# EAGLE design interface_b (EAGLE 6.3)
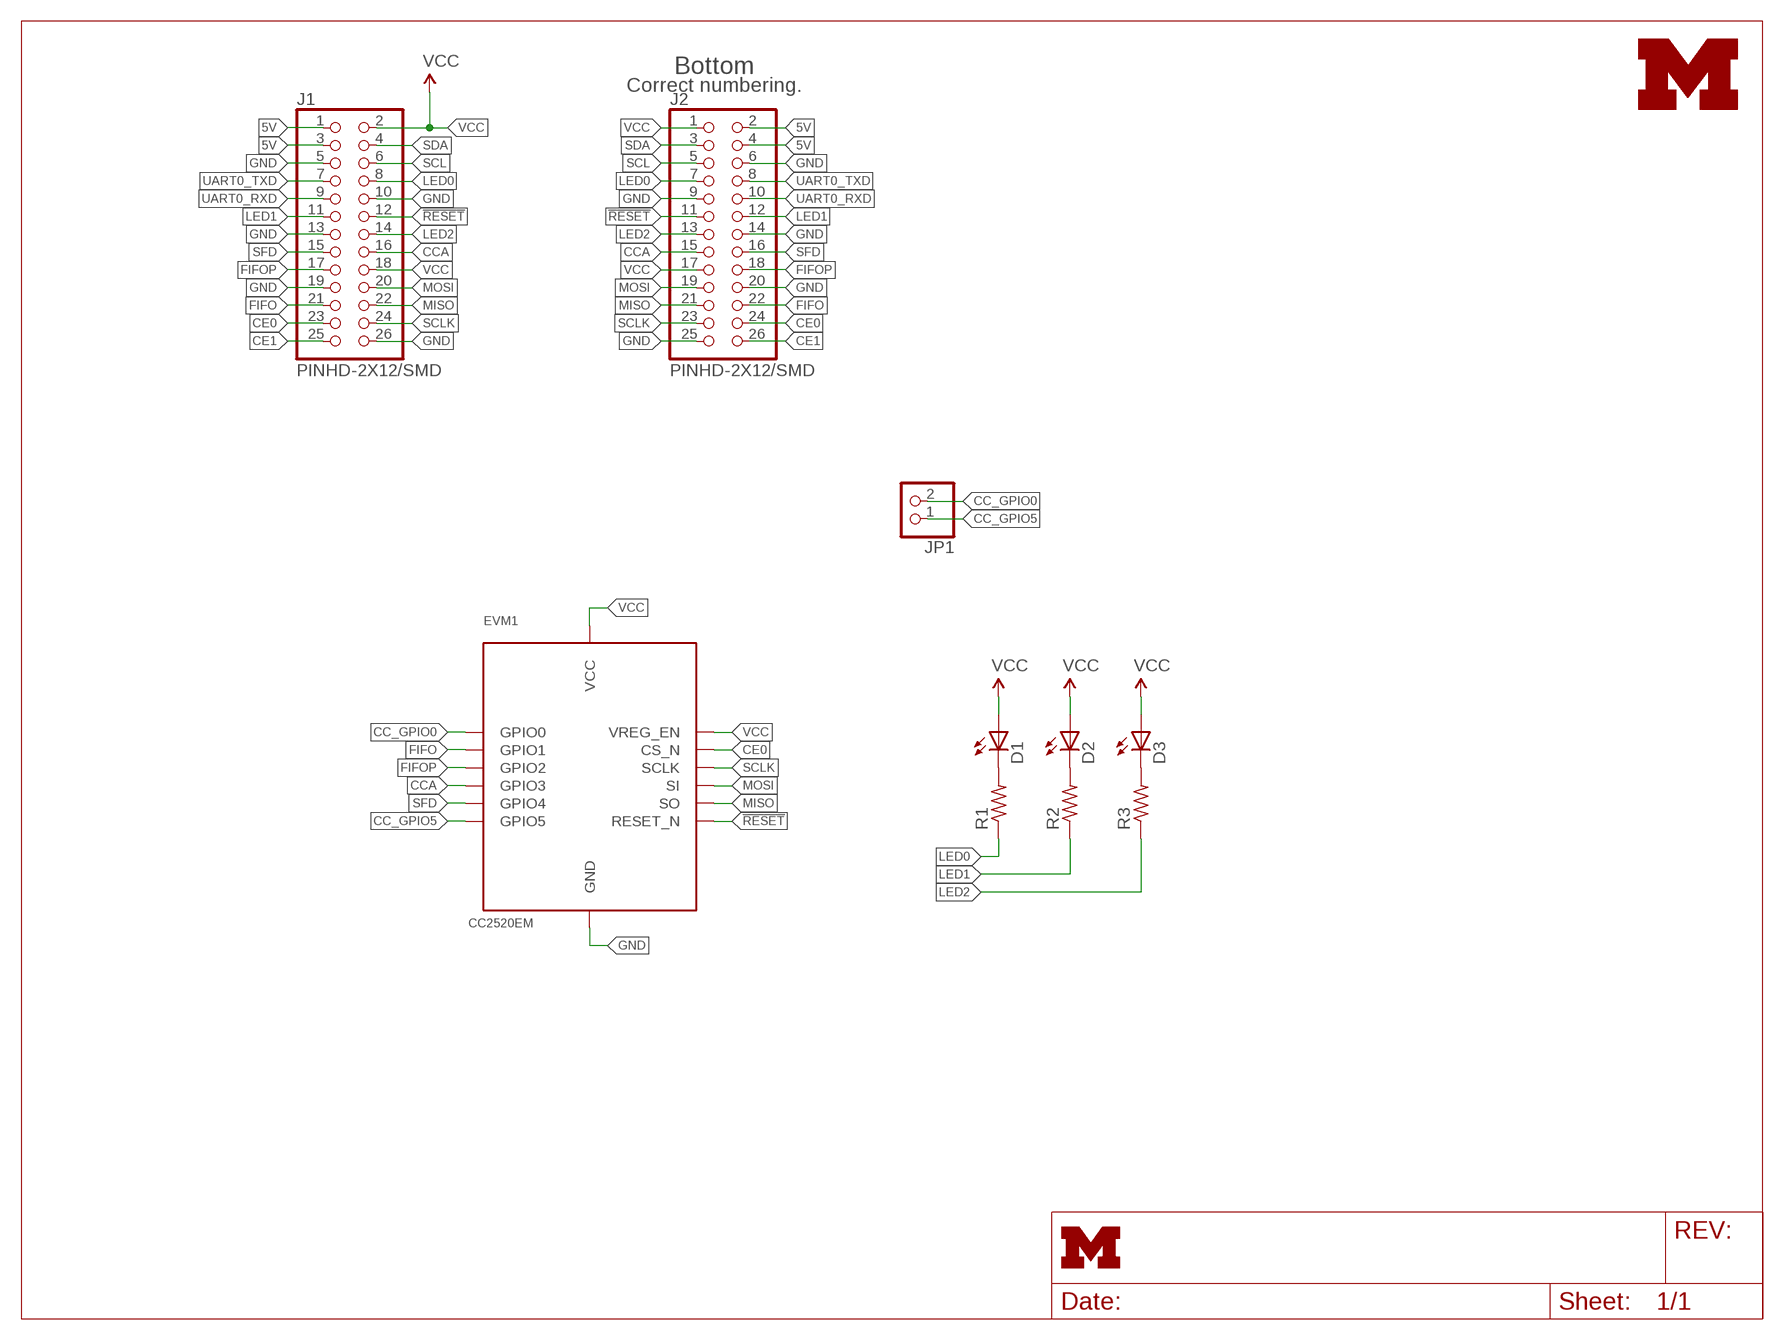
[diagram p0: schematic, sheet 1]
FRAME1 (LETTER_L): HEIGHT: 8.5in; WIDTH: 11in

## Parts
D1  LED0603  [LED-0603]
D2  LED0603  [LED-0603]
D3  LED0603  [LED-0603]
EVM1  CC2520EM  [TI_CC_EVM]
J1  PINHD-2X12/SMD  [2X13/SMD]
J2  PINHD-2X12/SMD  [2X13/SMD]
JP1  PINHD-1X2  [1X02]
R1  R-US_R0603  [R0603]
R2  R-US_R0603  [R0603]
R3  R-US_R0603  [R0603]
U$1  UMICH_SOLID_SMALL  [UMICH_SOLID_75MIL]

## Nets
5V: J1.1 J1.3 J2.2 J2.4
!RESET: EVM1.P2_15(RESET_N) J1.12 J2.11
CC_GPIO0: EVM1.P1_3(GPIO0) JP1.2
CC_GPIO5: EVM1.P2_19(GPIO5) JP1.1
CCA: EVM1.P1_12(GPIO3) J1.16 J2.15
CE0: EVM1.P1_14(CS_N) J1.23 J2.24
CE1: J1.25 J2.26
FIFO: EVM1.P1_7(GPIO1) J1.21 J2.22
FIFOP: EVM1.P1_9(GPIO2) J1.17 J2.18
GND: EVM1.P1_1(GND) EVM1.P1_19(GND) J1.5 J1.10 J1.13 J1.19 J1.26 J2.6 J2.9 J2.14 J2.20 J2.25
LED0: J1.8 J2.7 R1.1
LED1: J1.11 J2.12 R2.1
LED2: J1.14 J2.13 R3.1
MISO: EVM1.P1_20(SO) J1.22 J2.21
MOSI: EVM1.P1_18(SI) J1.20 J2.19
N$1: D1.C R1.2
N$2: D2.C R2.2
N$3: D3.C R3.2
SCL: J1.6 J2.5
SCLK: EVM1.P1_16(SCLK) J1.24 J2.23
SDA: J1.4 J2.3
SFD: EVM1.P2_18(GPIO4) J1.15 J2.16
UART0_RXD: J1.9 J2.10
UART0_TXD: J1.7 J2.8
VCC: D1.A D2.A D3.A EVM1.P1_10(VREG_EN) EVM1.P2_7(VCC) EVM1.P2_9(VCC) J1.2 J1.18 J2.1 J2.17

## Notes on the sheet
- Bottom
- Correct numbering.

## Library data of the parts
D1-D3 = SparkFun-LED:LED: LEDs
EVM1 = brouter:CC2520EM: CC2520 EVM http://ti.com/tool/cc2520em_refdes
J1 J2 = headers:PINHD-2X12/SMD: 23 pin 2 row smd 0.100 pitch header
JP1 = pinhead:PINHD-1X2: PIN HEADER
R1-R3 = rcl:R-US_: RESISTOR, American symbol
U$1 = logos:UMICH_SOLID

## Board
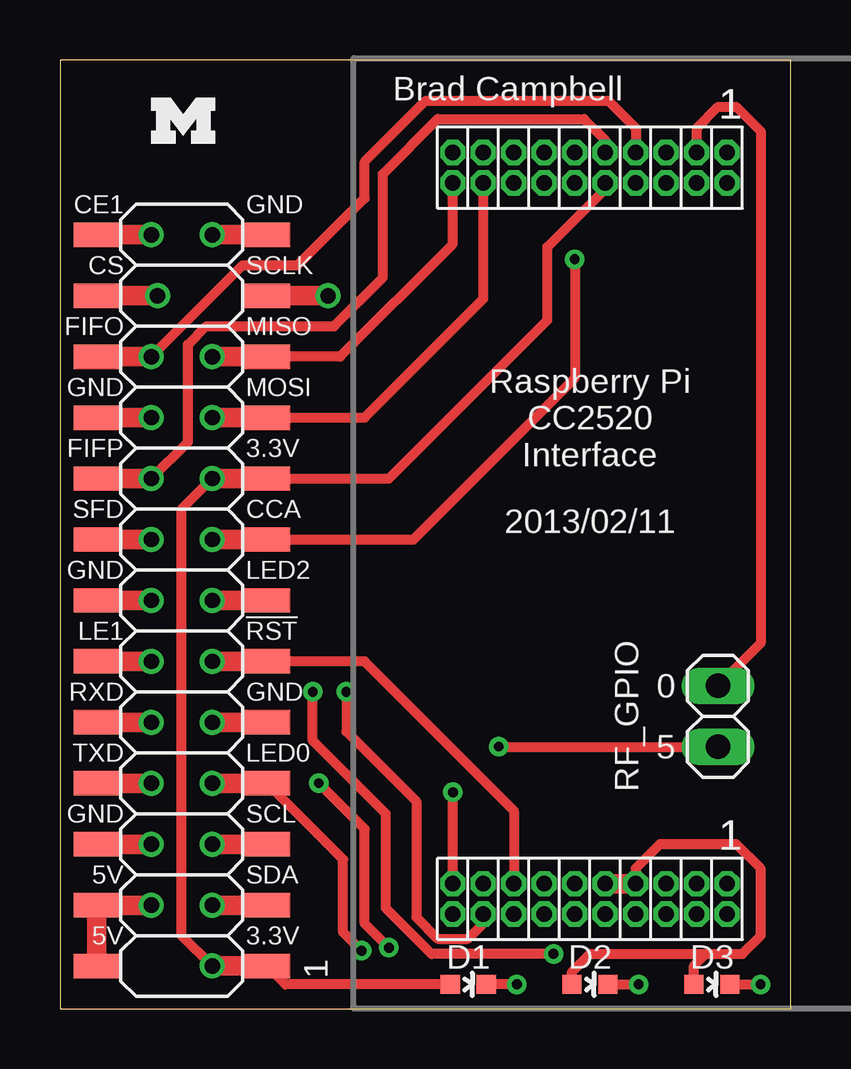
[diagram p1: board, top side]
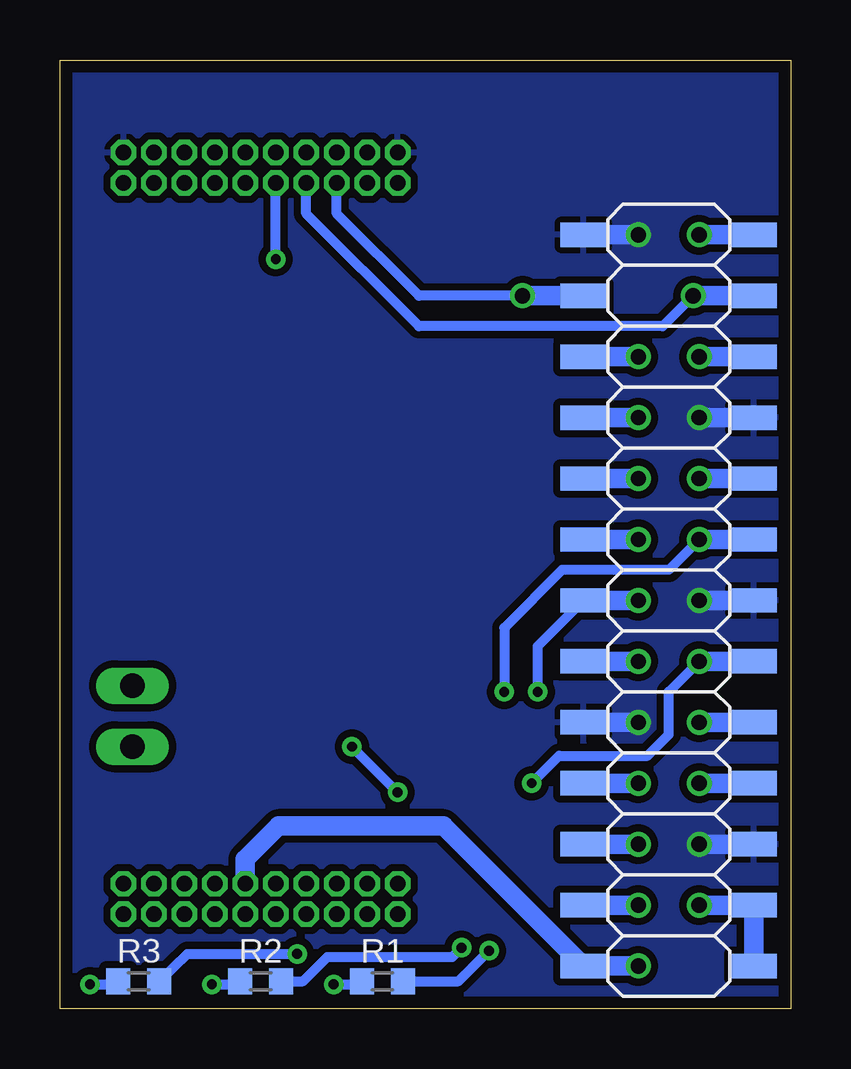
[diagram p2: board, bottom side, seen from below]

Size 30.46 x 39.55 mm. Coordinates in mm from the lower left corner, seen from the top.
Outline: 0,0 30.46,0 30.46,39.55 0,39.55 0,0
Copper layers (1*16): Top 0.0178mm / dielectric 59mil / Bottom 0.0178mm
Design rules "default *": minimum track width 6mil, minimum drill 14mil, track to track 6mil, track to pad 6mil, pad to pad 6mil, via to via 6mil, smd to smd 6mil, copper to edge 20mil, drill to drill 16mil, minimum pad ring 8mil, minimum via ring 8mil, stop-mask expansion 3mil, vias tented up to drill 25mil, thermal gap 10mil

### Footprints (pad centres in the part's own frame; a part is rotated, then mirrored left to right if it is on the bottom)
LED-0603 = smd 0.8 x 0.8: A 0,-0.75; C 0,0.75
TI_CC_EVM = drill 0.65 octagon: P1_1 5.715,15.875; P1_2 5.715,14.605; P1_3 4.445,15.875; P1_4 4.445,14.605; P1_5 3.175,15.875; P1_6 3.175,14.605; P1_7 1.905,15.875; P1_8 1.905,14.605; P1_9 0.635,15.875; P1_10 0.635,14.605; P1_11 -0.635,15.875; P1_12 -0.635,14.605; P1_13 -1.905,15.875; P1_14 -1.905,14.605; P1_15 -3.175,15.875; P1_16 -3.175,14.605; P1_17 -4.445,15.875; P1_18 -4.445,14.605; P1_19 -5.715,15.875; P1_20 -5.715,14.605; P2_1 5.715,-14.605; P2_2 5.715,-15.875; P2_3 4.445,-14.605; P2_4 4.445,-15.875; P2_5 3.175,-14.605; P2_6 3.175,-15.875; P2_7 1.905,-14.605; P2_8 1.905,-15.875; P2_9 0.635,-14.605; P2_10 0.635,-15.875; P2_11 -0.635,-14.605; P2_12 -0.635,-15.875; P2_13 -1.905,-14.605; P2_14 -1.905,-15.875; P2_15 -3.175,-14.605; P2_16 -3.175,-15.875; P2_17 -4.445,-14.605; P2_18 -4.445,-15.875; P2_19 -5.715,-14.605; P2_20 -5.715,-15.875
2X13/SMD = smd 1.016 x 1.905: 1 -15.24,-3.556; 2 -15.24,3.556; 3 -12.7,-3.556; 4 -12.7,3.556; 5 -10.16,-3.556; 6 -10.16,3.556; 7 -7.62,-3.556; 8 -7.62,3.556; 9 -5.08,-3.556; 10 -5.08,3.556; 11 -2.54,-3.556; 12 -2.54,3.556; 13 0,-3.556; 14 0,3.556; 15 2.54,-3.556; 16 2.54,3.556; 17 5.08,-3.556; 18 5.08,3.556; 19 7.62,-3.556; 20 7.62,3.556; 21 10.16,-3.556; 22 10.16,3.556; 23 12.7,-3.556; 24 12.7,3.556; 25 15.24,-3.556; 26 15.24,3.556
1X02 = drill 1.016 long: 1 -1.27,0; 2 1.27,0
R0603 = smd 1 x 1.1: 1 -0.85,0; 2 0.85,0

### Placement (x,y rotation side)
D1  17.02,1.02 270 top
D2  22.1,1.02 270 top
D3  27.18,1.02 270 top
EVM1  22.1,19.81 0 top
J1  5.08,17.02 90 bottom
J2  5.08,17.02 90 top
JP1  27.43,12.19 90 top
R1  17.02,1.14 180 bottom
R2  22.1,1.14 180 bottom
R3  27.18,1.14 180 bottom
U$1  3.81,36.07 0 top

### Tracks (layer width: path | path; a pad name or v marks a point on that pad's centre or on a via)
5V  (via drill 0.64)
  Top 0.813: J2.2 J2.4 v3.81,4.32
  Bottom 0.813: v3.81,4.32 J2.4 J2.2
!RESET  (via drill 0.64)
  Top 0.406: J2.11 12.7,14.48 18.92,8.26 EVM1.P2_15
  Top 0.813: J2.11 v6.35,14.48
  Bottom 0.813: v6.35,14.48 J2.11
CC_GPIO0
  Top 0.406: EVM1.P1_3 26.54,36.7 27.43,37.59 28.19,37.59 29.21,36.58 29.21,15.24 JP1.2
CC_GPIO5  (via drill 0.41)
  Top 0.406: EVM1.P2_19 v16.38,9.02 | v18.29,10.92 JP1.1
  Bottom 0.406: v16.38,9.02 v18.29,10.92
CCA  (via drill 0.41, 0.64)
  Top 0.406: J1.16 14.73,19.56 21.46,26.29 v21.46,31.24
  Top 0.813: J1.16 v6.35,19.56
  Bottom 0.406: v21.46,31.24 EVM1.P1_12
  Bottom 0.813: v6.35,19.56 J1.16
CE0  (via drill 0.64)
  Top 0.813: v4.06,29.72 J2.24
  Bottom 0.406: v4.06,29.72 5.33,28.45 15.49,28.45 20.19,33.15 EVM1.P1_14
  Bottom 0.813: J2.24 v4.06,29.72
CE1  (via drill 0.64)
  Top 0.813: J2.26 v3.81,32.26
  Bottom 0.813: v3.81,32.26 J2.26
FIFO  (via drill 0.64)
  Top 0.406: EVM1.P1_7 24,36.7 22.86,37.85 15.24,37.85 12.7,35.31 12.7,33.78 9.91,30.99 7.62,30.99 v3.81,27.18
  Top 0.813: v3.81,27.18 J1.21
  Bottom 0.813: v3.81,27.18 J1.21
FIFOP  (via drill 0.64)
  Top 0.406: v3.81,22.1 5.33,23.62 5.33,27.69 6.1,28.45 11.43,28.45 13.46,30.48 13.46,34.8 15.75,37.08 21.84,37.08 22.73,36.2 EVM1.P1_9
  Top 0.813: J1.17 v3.81,22.1
  Bottom 0.813: v3.81,22.1 J1.17
GND  (via drill 0.64)
  Top 0.813: v6.35,32.26 J2.25 | v6.35,11.94 J2.9 | J2.14 v3.81,17.02 | J2.6 v3.81,6.86 | J2.20 v3.81,24.64
  Bottom 0.813: J2.25 v6.35,32.26 | J2.9 v6.35,11.94 | v3.81,17.02 J2.14 | v3.81,6.86 J2.6 | v3.81,24.64 J2.20
  pour Bottom (isolate 0.305): 0,39.62 30.48,39.62 30.48,0 0,0
LED0  (via drill 0.41, 0.64)
  Top 0.406: v12.57,2.41 11.81,3.17 11.81,6.22 J2.7
  Top 0.813: J2.7 v6.35,9.4
  Bottom 0.406: R1.1 13.84,1.14 v12.57,2.41
  Bottom 0.813: v6.35,9.4 J2.7
LED1  (via drill 0.41, 0.64)
  Top 0.406: v13.72,2.54 12.7,3.56 12.7,7.49 v10.79,9.4
  Top 0.813: v3.81,14.48 J2.12
  Bottom 0.406: v13.72,2.54 14.1,2.16 19.3,2.16 20.32,1.14 R2.1 | v10.79,9.4 9.65,10.54 5.97,10.54 5.08,11.43 5.08,13.21 v3.81,14.48
  Bottom 0.813: J2.12 v3.81,14.48
LED2  (via drill 0.41, 0.64)
  Top 0.406: v20.57,2.29 15.49,2.29 13.59,4.19 13.59,8.13 10.54,11.18 v10.54,13.21
  Top 0.813: v6.35,17.02 J2.13
  Bottom 0.406: R3.1 25.15,2.29 v20.57,2.29 | v10.54,13.21 10.54,15.11 J2.13
  Bottom 0.813: J2.13 v6.35,17.02
MISO  (via drill 0.64)
  Top 0.406: J2.21 11.68,27.18 16.38,31.88 EVM1.P1_20
  Top 0.813: J2.21 v6.35,27.18
  Bottom 0.813: v6.35,27.18 J2.21
MOSI  (via drill 0.64)
  Top 0.406: J2.19 12.7,24.64 17.65,29.59 EVM1.P1_18
  Top 0.813: J2.19 v6.35,24.64
  Bottom 0.813: v6.35,24.64 J2.19
N$1  (via drill 0.41)
  Top 0.406: v19.05,1.02 D1.C
  Bottom 0.406: 17.78,1.27 R1.2 18,1.02 v19.05,1.02
N$2  (via drill 0.41)
  Top 0.406: D2.C v24.13,1.02
  Bottom 0.406: 22.85,1.27 R2.2 23.07,1.02 v24.13,1.02
N$3  (via drill 0.41)
  Top 0.406: D3.C v29.21,1.02
  Bottom 0.406: v29.21,1.02 28.16,1.02 R3.2
SCL  (via drill 0.64)
  Top 0.813: J2.5 v6.35,6.86
  Bottom 0.813: v6.35,6.86 J2.5
SCLK  (via drill 0.64)
  Top 0.813: v11.18,29.72 J2.23
  Bottom 0.406: 9.65,29.72 J2.23 | v11.18,29.72 15.49,29.72 18.92,33.15 EVM1.P1_16
  Bottom 0.813: v11.18,29.72 9.65,29.72
SDA  (via drill 0.64)
  Top 0.813: v6.35,4.32 J2.3
  Bottom 0.813: J2.3 v6.35,4.32
SFD  (via drill 0.41, 0.64)
  Top 0.406: v11.94,13.21 11.94,11.56 14.86,8.64 14.86,3.81 15.75,2.92 17.02,2.92 17.65,3.56 EVM1.P2_18
  Top 0.813: v3.81,19.56 J1.15
  Bottom 0.406: v3.81,19.56 5.08,18.29 9.53,18.29 11.94,15.88 v11.94,13.21
  Bottom 0.813: J1.15 v3.81,19.56
UART0_RXD  (via drill 0.64)
  Top 0.813: J2.10 v3.81,11.94
  Bottom 0.813: v3.81,11.94 J2.10
UART0_TXD  (via drill 0.64)
  Top 0.813: v3.81,9.4 J2.8
  Bottom 0.813: J2.8 v3.81,9.4
VCC  (via drill 0.64)
  Top 0.406: v6.35,1.78 5.08,3.05 5.08,20.83 v6.35,22.1 | J2.17 13.72,22.1 20.32,28.7 20.32,31.75 22.73,34.16 EVM1.P1_10 | D1.A 9.4,1.02 J2.1 | D3.A 26.43,1.79 26.92,2.29 | 26.92,2.29 28.45,2.29 29.21,3.05 29.21,5.84 28.19,6.86 25.02,6.86 24,5.84 EVM1.P2_7 | D2.A 21.35,1.54 22.1,2.29 26.92,2.29
  Top 0.813: EVM1.P2_7 EVM1.P2_9 | J2.1 v6.35,1.78 | v6.35,22.1 J2.17
  Bottom 0.813: v6.35,22.1 J2.17 | EVM1.P2_9 22.73,6.22 21.34,7.62 14.48,7.62 J2.1 v6.35,1.78

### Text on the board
tPlace: Brad Campbell | CE1 | GND | CS | SCLK | FIFO | MISO | GND | MOSI | FIFP | 3.3V | Raspberry Pi / CC2520 / Interface | SFD | CCA | 2013/02/11 | GND | LED2 | LE1 | !RST | RXD | GND | 0 | RF_GPIO | TXD | LED0 | 5 | GND | SCL | 5V | SDA | 5V | 3.3V | 1

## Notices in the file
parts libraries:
SparkFun-LED: Licensing: CC v3.0 Share-Alike You are welcome to use this library for commercial purposes.
